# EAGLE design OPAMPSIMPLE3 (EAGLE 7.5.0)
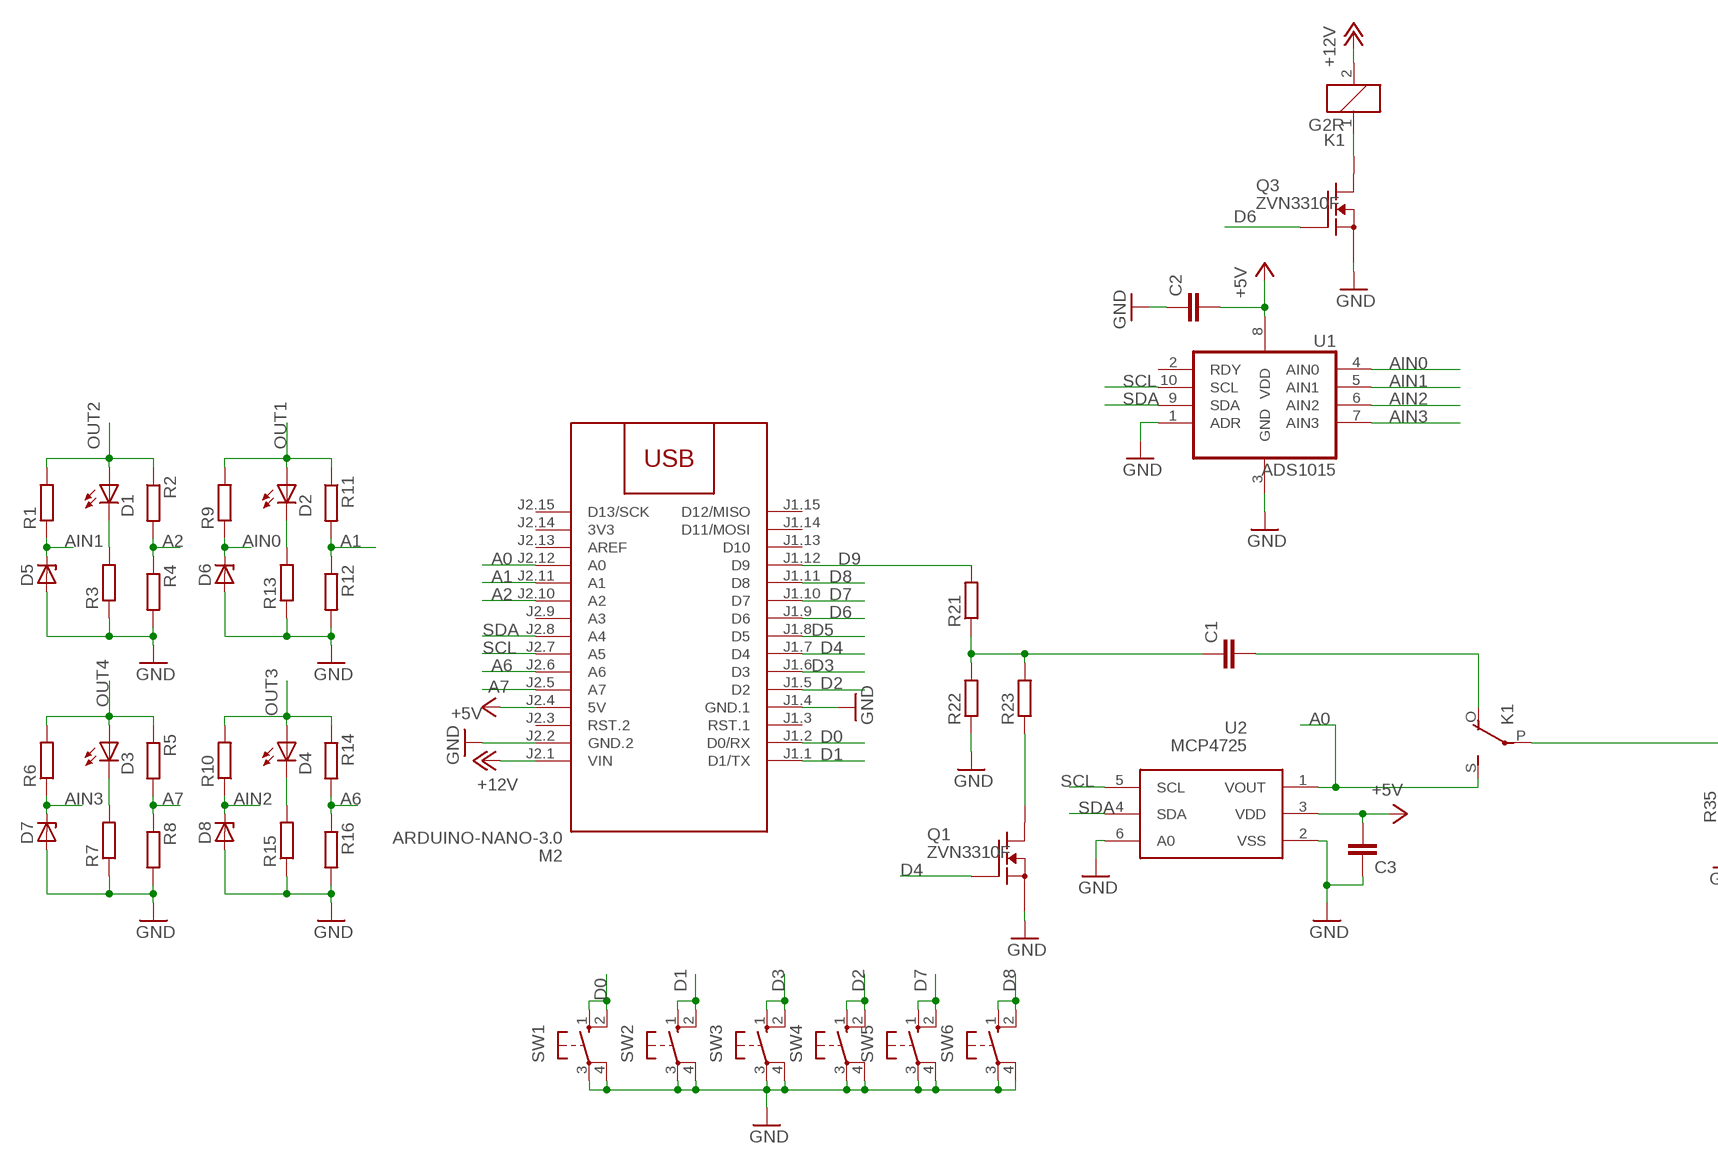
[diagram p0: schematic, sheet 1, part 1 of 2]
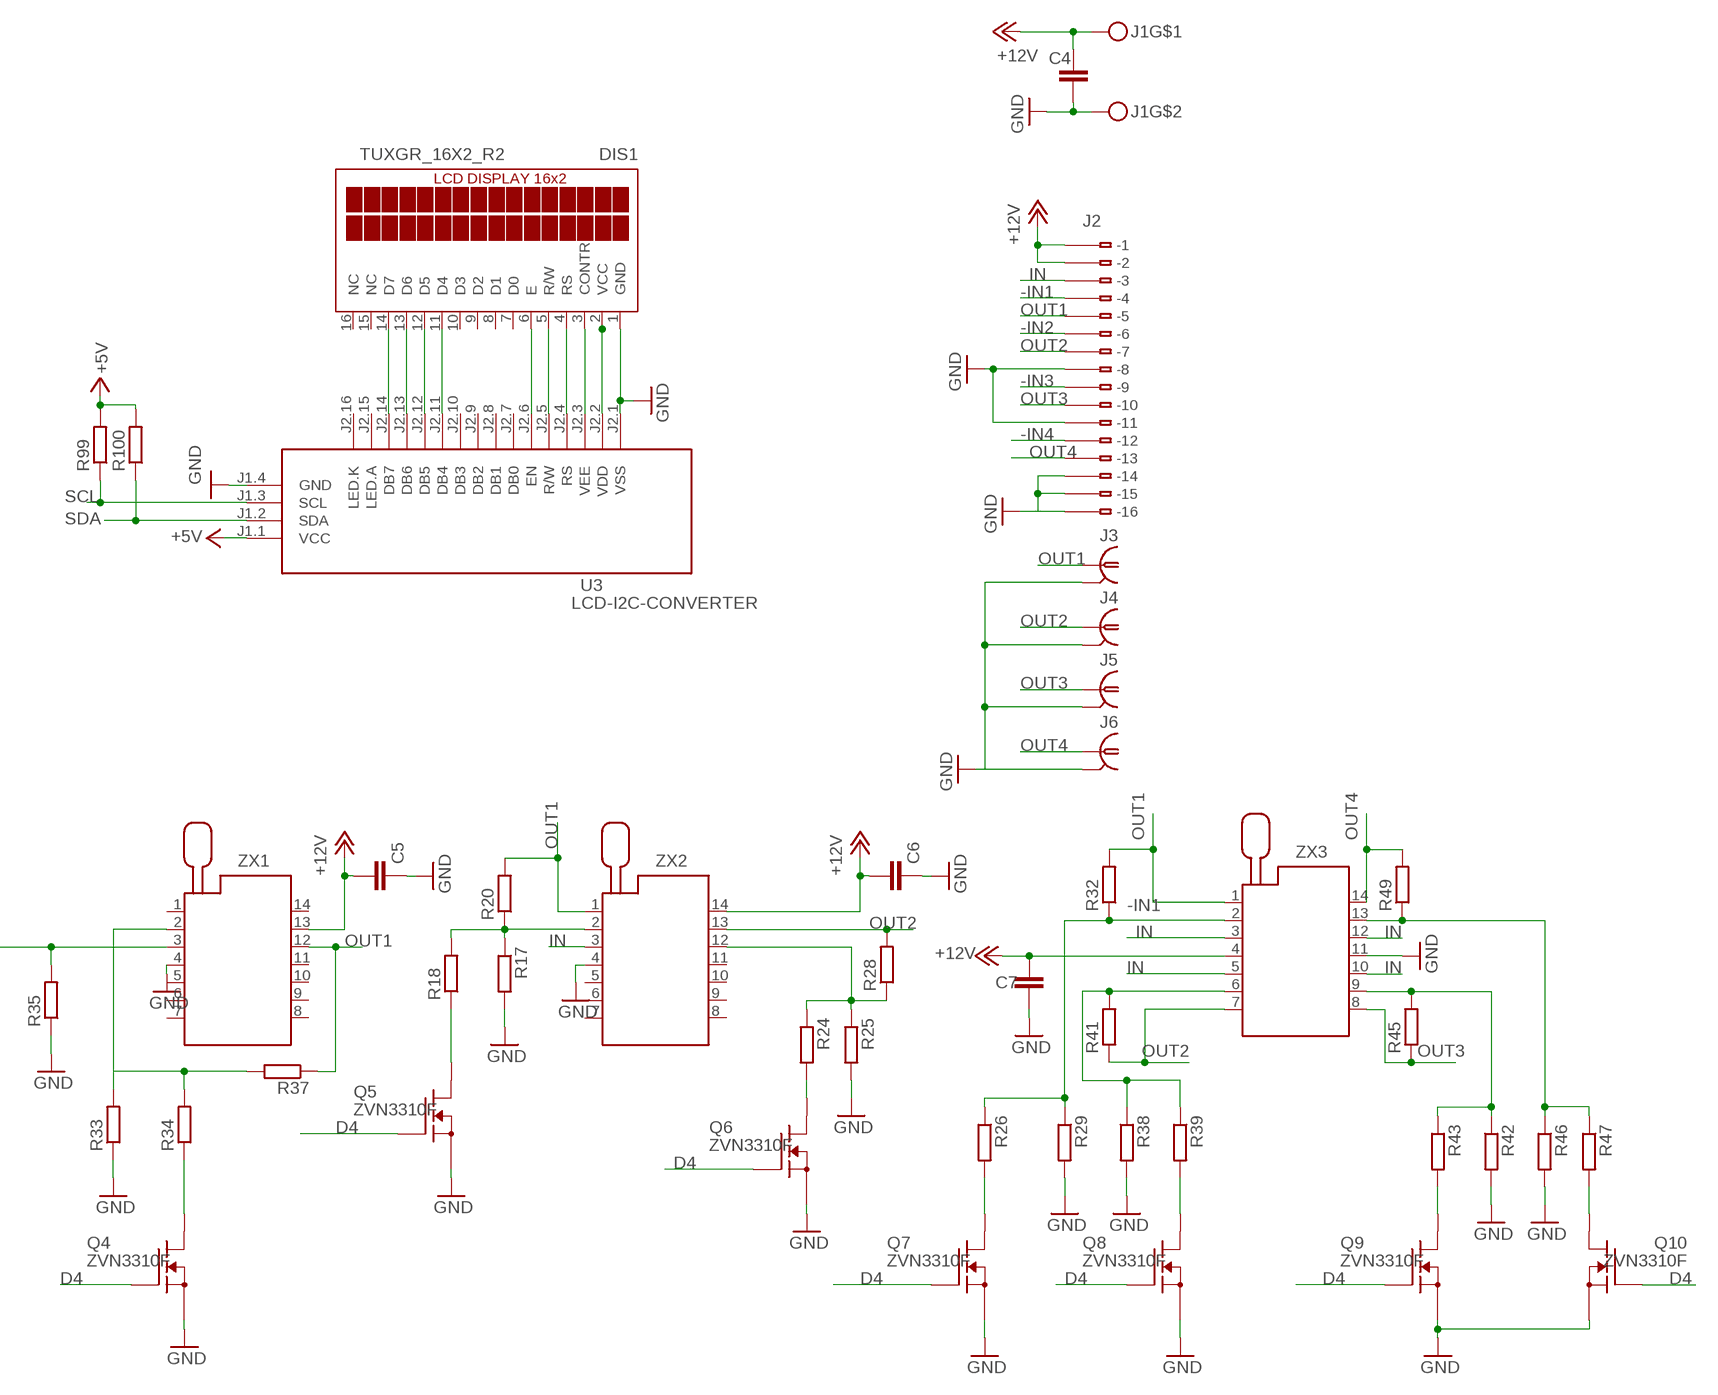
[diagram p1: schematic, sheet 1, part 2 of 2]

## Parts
C1  C-EUC1206  [C1206]
C2  C-EUC1206  [C1206]
C3  C-EUC1206  [C1206]
C4  C-EUC1206  [C1206]
C5  C-EUC1206  [C1206]
C6  C-EUC1206  [C1206]
C7  C-EUC1206  [C1206]
D1  LED5MM  [LED5MM]
D2  LED5MM  [LED5MM]
D3  LED5MM  [LED5MM]
D4  LED5MM  [LED5MM]
D5  BZX84CSMD  [TO236]
D6  BZX84CSMD  [TO236]
D7  BZX84CSMD  [TO236]
D8  BZX84CSMD  [TO236]
DIS1  TUXGR_16X2_R2  [TUXGR_16X2_R2]
J1  MKDSN1,5-2-5,08  [MKDSN1,5-2-5,08]
J2  233-116  [233-116]
J3  1-227161-0  [AMP_227161]
J4  1-227161-0  [AMP_227161]
J5  1-227161-0  [AMP_227161]
J6  1-227161-0  [AMP_227161]
K1  G2R  [G2R]
M2  ARDUINO-NANO-3.0  [ARDUINO-NANO-3.0]
Q1  ZVN3310F  BSS138  [SOT23]
Q3  ZVN3310F  BSS138  [SOT23]
Q4  ZVN3310F  BSS138  [SOT23]
Q5  ZVN3310F  BSS138  [SOT23]
Q6  ZVN3310F  BSS138  [SOT23]
Q7  ZVN3310F  BSS138  [SOT23]
Q8  ZVN3310F  BSS138  [SOT23]
Q9  ZVN3310F  BSS138  [SOT23]
Q10  ZVN3310F  BSS138  [SOT23]
R1  R-EU_R1206  [R1206]
R2  R-EU_R1206  [R1206]
R3  R-EU_R1206  [R1206]
R4  R-EU_R1206  [R1206]
R5  R-EU_R1206  [R1206]
R6  R-EU_R1206  [R1206]
R7  R-EU_R1206  [R1206]
R8  R-EU_R1206  [R1206]
R9  R-EU_R1206  [R1206]
R10  R-EU_R1206  [R1206]
R11  R-EU_R1206  [R1206]
R12  R-EU_R1206  [R1206]
R13  R-EU_R1206  [R1206]
R14  R-EU_R1206  [R1206]
R15  R-EU_R1206  [R1206]
R16  R-EU_R1206  [R1206]
R17  R-EU_R1206  [R1206]
R18  R-EU_R1206  [R1206]
R20  R-EU_R1206  [R1206]
R21  R-EU_R1206  [R1206]
R22  R-EU_R1206  [R1206]
R23  R-EU_R1206  [R1206]
R24  R-EU_R1206  [R1206]
R25  R-EU_R1206  [R1206]
R26  R-EU_R1206  [R1206]
R28  R-EU_R1206  [R1206]
R29  R-EU_R1206  [R1206]
R32  R-EU_R1206  [R1206]
R33  R-EU_R1206  [R1206]
R34  R-EU_R1206  [R1206]
R35  R-EU_R1206  [R1206]
R37  R-EU_R1206  [R1206]
R38  R-EU_R1206  [R1206]
R39  R-EU_R1206  [R1206]
R41  R-EU_R1206  [R1206]
R42  R-EU_R1206  [R1206]
R43  R-EU_R1206  [R1206]
R45  R-EU_R1206  [R1206]
R46  R-EU_R1206  [R1206]
R47  R-EU_R1206  [R1206]
R49  R-EU_R1206  [R1206]
R99  R-EU_R1206  [R1206]
R100  R-EU_R1206  [R1206]
SW1  40-XX  [B3F-40XX]
SW2  40-XX  [B3F-40XX]
SW3  40-XX  [B3F-40XX]
SW4  40-XX  [B3F-40XX]
SW5  40-XX  [B3F-40XX]
SW6  40-XX  [B3F-40XX]
U1  ADS1015  [ADS1015]
U2  MCP4725  [SOT23-6]
U3  LCD-I2C-CONVERTER  [LCD-I2C-CONVERTER]
ZX1  214-3339-00-0602J  [214-3339-00-0602J]
ZX2  214-3339-00-0602J  [214-3339-00-0602J]
ZX3  214-3339-00-0602J  [214-3339-00-0602J]

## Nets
+5V: C2.2 C3.2 M2.J2.4(5V) R99.2 R100.2 U1.8(VDD) U2.3(VDD) U3.J1.1(VCC)
+12V: C4.1 C5.2 C6.2 C7.1 J1.1 J2.B1(B-1) J2.B2(B-2) K1.2 M2.J2.1(VIN) ZX1.13 ZX2.14 ZX3.4
-IN1: J2.B4(B-4) R26.1 R29.1 R32.1 ZX3.2
-IN2: J2.B6(B-6) R38.1 R39.1 R41.2 ZX3.6
-IN3: J2.B9(B-9) R42.1 R43.1 R45.2 ZX3.9
-IN4: J2.B12(B-12) R46.1 R47.1 R49.1 ZX3.13
A0: K1.S(2:S) M2.J2.12(A0) U2.1(VOUT)
A1: M2.J2.11(A1) R11.2 R12.1
A2: M2.J2.10(A2) R2.2 R4.1
A6: M2.J2.6(A6) R14.2 R16.1
A7: M2.J2.5(A7) R5.2 R8.1
AIN0: D6.C R9.1 U1.4(AIN0)
AIN1: D5.C R1.1 U1.5(AIN1)
AIN2: D8.C R10.1 U1.6(AIN2)
AIN3: D7.C R6.1 U1.7(AIN3)
D0: M2.J1.2(D0/RX) SW1.1(S) SW1.2(S1)
D1: M2.J1.1(D1/TX) SW2.1(S) SW2.2(S1)
D2: M2.J1.5(D2) SW4.1(S) SW4.2(S1)
D3: M2.J1.6(D3) SW3.1(S) SW3.2(S1)
D4: M2.J1.7(D4) Q1.3(G) Q4.3(G) Q5.3(G) Q6.3(G) Q7.3(G) Q8.3(G) Q9.3(G) Q10.3(G)
D5: M2.J1.8(D5)
D6: M2.J1.9(D6) Q3.3(G)
D7: M2.J1.10(D7) SW5.1(S) SW5.2(S1)
D8: M2.J1.11(D8) SW6.1(S) SW6.2(S1)
D9: M2.J1.12(D9) R21.2
GND: C2.1 C3.1 C4.2 C5.1 C6.1 C7.2 D5.A D6.A D7.A D8.A DIS1.1(GND) J1.2 J2.B8(B-8) J2.B11(B-11) J2.B14(B-14) J2.B15(B-15) J2.B16(B-16) J3.2 J4.2 J5.2 J6.2 M2.J1.4(GND.1) M2.J2.2(GND.2) Q1.1(S) Q3.1(S) Q4.1(S) Q5.1(S) Q6.1(S) Q7.1(S) Q8.1(S) Q9.1(S) Q10.1(S) R3.1 R4.2 R7.1 R8.2 R12.2 R13.1 R15.1 R16.2 R17.2 R22.1 R25.2 R29.2 R33.1 R35.1 R38.2 R42.2 R46.2 SW1.3(P) SW1.4(P1) SW2.3(P) SW2.4(P1) SW3.3(P) SW3.4(P1) SW4.3(P) SW4.4(P1) SW5.3(P) SW5.4(P1) SW6.3(P) SW6.4(P1) U1.1(ADR) U1.3(GND) U2.2(VSS) U2.6(A0) U3.J1.4(GND) U3.J2.1(VSS) ZX1.4 ZX2.4 ZX3.11
IN: J2.B3(B-3) K1.P(2:P) R35.2 ZX1.3 ZX2.3 ZX3.3 ZX3.5 ZX3.10 ZX3.12
N$1: DIS1.14(D7) U3.J2.14(DB7)
N$2: DIS1.13(D6) U3.J2.13(DB6)
N$3: DIS1.12(D5) U3.J2.12(DB5)
N$4: DIS1.11(D4) U3.J2.11(DB4)
N$5: DIS1.6(E) U3.J2.6(EN)
N$6: DIS1.5(R/W) U3.J2.5(R/W)
N$7: DIS1.4(RS) U3.J2.4(RS)
N$8: C1.1 R21.1 R22.2 R23.2
N$10: DIS1.3(CONTR) U3.J2.3(VEE)
N$11: DIS1.2(VCC) U3.J2.2(VDD)
N$12: Q8.2(D) R39.2
N$13: R17.1 R18.2 R20.1 ZX2.2
N$14: K1.1 Q3.2(D)
N$15: R33.2 R34.2 R37.2 ZX1.2
N$16: C1.2 K1.O(2:O)
N$17: Q4.2(D) R34.1
N$18: Q5.2(D) R18.1
N$19: Q6.2(D) R24.2
N$20: D1.K(C) R3.2
N$21: Q7.2(D) R26.2
N$23: D2.K(C) R13.2
N$24: Q10.2(D) R47.2
N$25: Q9.2(D) R43.2
N$26: D3.K(C) R7.2
N$27: Q1.2(D) R23.1
N$29: D4.K(C) R15.2
N$32: R24.1 R25.1 R28.1 ZX2.12
OUT1: D2.A J2.B5(B-5) J3.1 R9.2 R11.1 R20.2 R32.2 R37.1 ZX1.12 ZX2.1 ZX3.1
OUT2: D1.A J2.B7(B-7) J4.1 R1.2 R2.1 R28.2 R41.1 ZX2.13 ZX3.7
OUT3: D4.A J2.B10(B-10) J5.1 R10.2 R14.1 R45.1 ZX3.8
OUT4: D3.A J2.B13(B-13) J6.1 R5.1 R6.2 R49.2 ZX3.14
SCL: M2.J2.7(A5) R99.1 U1.10(SCL) U2.5(SCL) U3.J1.3(SCL)
SDA: M2.J2.8(A4) R100.1 U1.9(SDA) U2.4(SDA) U3.J1.2(SDA)
Unconnected: DIS1.7(D0) DIS1.8(D1) DIS1.9(D2) DIS1.10(D3) DIS1.15(NC) DIS1.16(NC) J2.A1(-1) J2.A2(-2) J2.A3(-3) J2.A4(-4) J2.A5(-5) J2.A6(-6) J2.A7(-7) J2.A8(-8) J2.A9(-9) J2.A10(-10) J2.A11(-11) J2.A12(-12) J2.A13(-13) J2.A14(-14) J2.A15(-15) J2.A16(-16) M2.J1.3(RST.1) M2.J1.13(D10) M2.J1.14(D11/MOSI) M2.J1.15(D12/MISO) M2.J2.3(RST.2) M2.J2.9(A3) M2.J2.13(AREF) M2.J2.15(D13/SCK) U1.2(RDY) U3.J2.7(DB0) U3.J2.8(DB1) U3.J2.9(DB2) U3.J2.10(DB3) U3.J2.15(LED.A) U3.J2.16(LED.K) ZX1.1 ZX1.5 ZX1.6 ZX1.7 ZX1.8 ZX1.9 ZX1.10 ZX1.11 ZX1.14 ZX2.5 ZX2.6 ZX2.7 ZX2.8 ZX2.9 ZX2.10 ZX2.11

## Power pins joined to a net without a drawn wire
3V3: M2.J2.14(3V3)

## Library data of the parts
C1-C7 = rcl:C-EU: CAPACITOR, European symbol
D1-D4 = led:LED: LED
D5-D8 = diode:BZX84CSMD: Z DIODE
DIS1 = display-lcd:TUXGR_16X2_R2: Tuxgraphics LCD display 16x2 characters reflective, without background light Source: tuxgr_12x2_r2.pdf; OC_FARNELL: unknown; OC_NEWARK: unknown
J1 = con-phoenix-508:MKDSN1,5-2-5,08
J2 = con-wago:233-116: WAGO Cage Clamp; MPN: 233-116; OC_FARNELL: unknown; OC_NEWARK: 28K9054
J3-J6 = con-coax:?227161*: JACK, RIGHT ANGLE, 50 OHM, PCB, BNC; MF: TYCO ELECTRONICS; MPN: 1-227161; OC_FARNELL: unknown; OC_NEWARK: 33B3200
K1 = relay:G2R: RELAY 1 x switch, Omron; OC_FARNELL: 1569185; OC_NEWARK: unknown
M2 = diy-modules:ARDUINO-NANO-3.0: Arduino Nano 3.0 and compatible devices More details available here: https://www.arduino.cc/en/Main/ArduinoBoardNano Click here to find device on ebay.com
Q1 Q3-Q10 = transistor-fet:BSS138
R1-R18 R20-R26 R28 R29 R32-R35 R37-R39 R41-R43 R45-R47 R49 R99 R100 = rcl:R-EU_: RESISTOR, European symbol
SW1-SW6 = switch-omron:40-XX: OMRON SWITCH; MF: OMRON COMPONENTS USA; MPN: B3F-4000; OC_FARNELL: 176434; OC_NEWARK: 36K3105
U1 = burr-brown:ADS1015: 12BIT I2C DAC
U2 = linear:MCP4725
U3 = diy-modules:LCD-I2C-CONVERTER: I2C Bus to 4-Bit Parallel LCD Interface with LED backlight driver
ZX1-ZX3 = con-3m:214-3339-00-0602J: Zero Insertion Force Socked Source: http://www.3M.com/ehpd; MF: 3M; MPN: 214-3339-00-0602J; OC_FARNELL: 1247151; OC_NEWARK: 85K7793

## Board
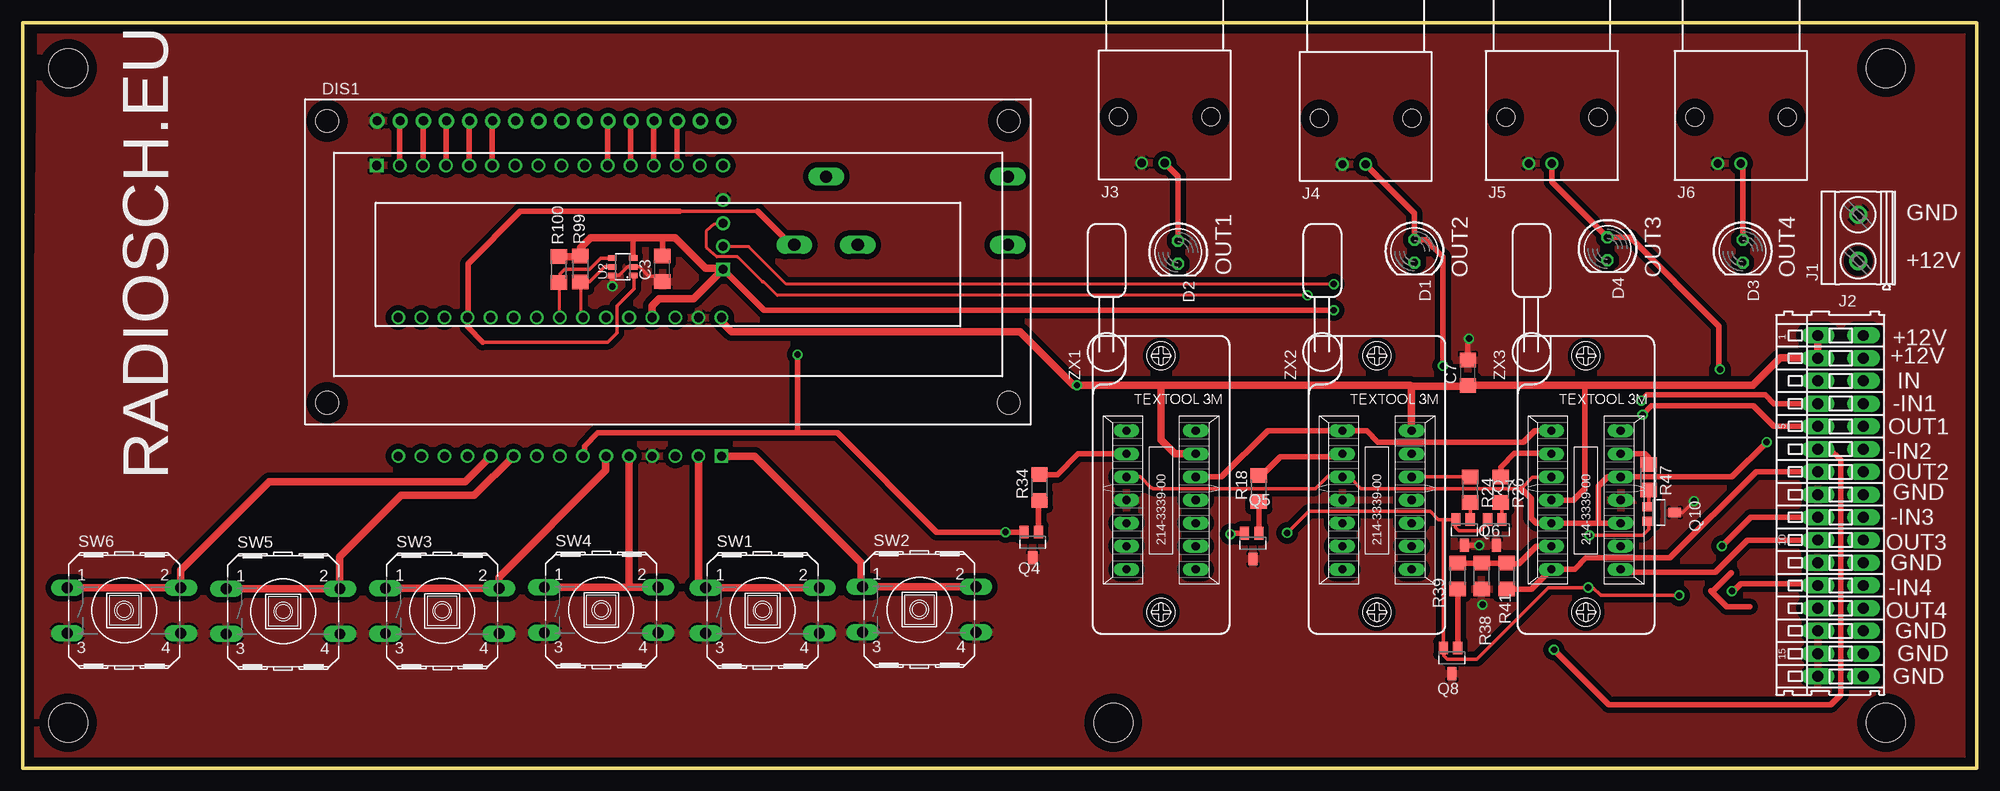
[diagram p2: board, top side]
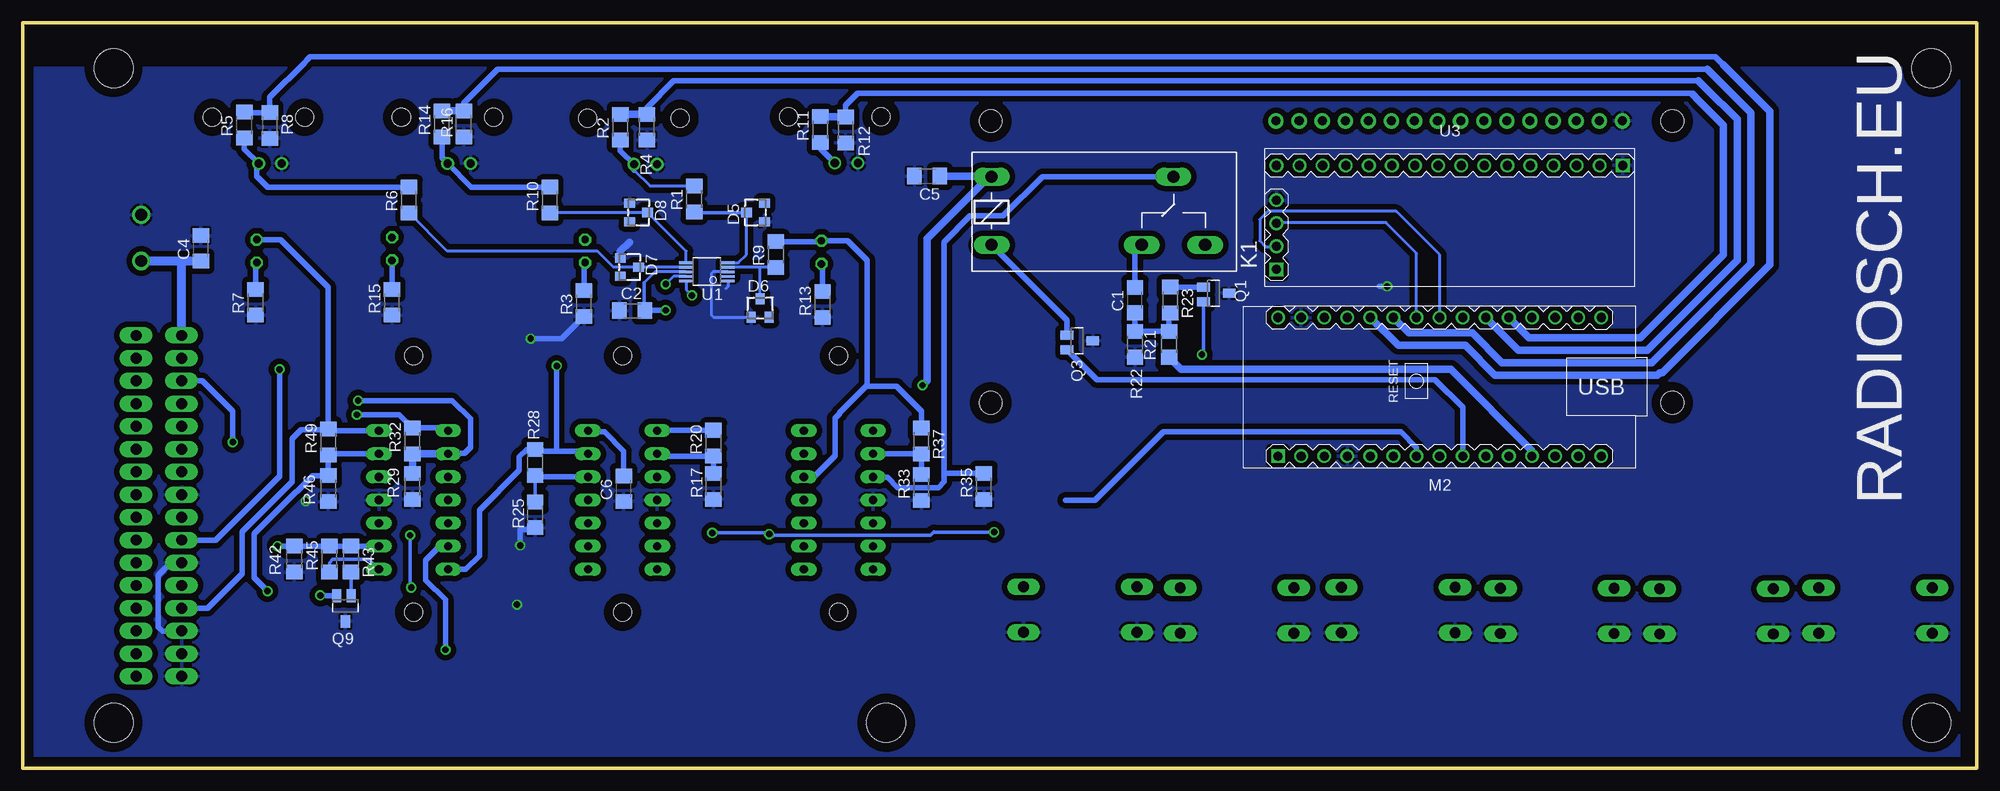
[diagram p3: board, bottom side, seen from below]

Size 215 x 82 mm. Coordinates in mm from the lower left corner, seen from the top.
Outline: 0,0 215,0 215,82 0,82 0,0
Copper layers (1*16): Top 0.035mm / dielectric 1.5mm / Bottom 0.035mm
Design rules "default": minimum track width 10mil, minimum drill 24mil, track to track 8mil, track to pad 8mil, pad to pad 8mil, via to via 8mil, smd to smd 8mil, copper to edge 40mil, drill to drill 8mil, minimum pad ring 10mil, minimum via ring 8mil, stop-mask expansion 4mil, vias tented up to drill 0mil, thermal gap 10mil
Holes 4.3 mm at 5,77 5,5 120,5 205,5 205,77

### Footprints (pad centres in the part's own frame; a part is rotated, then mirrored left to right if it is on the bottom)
C1206 = smd 1.6 x 1.8: 1 -1.4,0; 2 1.4,0
LED5MM = drill 0.813 octagon: A -1.27,0; K 1.27,0
TO236 = smd 1 x 1.2: A -1,-1; C 0,1; NC 1,-1
TUXGR_16X2_R2 = drill 1 pad 1.676: 1 -32,15.5; 2 -29.46,15.5; 3 -26.92,15.5; 4 -24.38,15.5; 5 -21.84,15.5; 6 -19.3,15.5; 7 -16.76,15.5; 8 -14.22,15.5; 9 -11.68,15.5; 10 -9.14,15.5; 11 -6.6,15.5; 12 -4.06,15.5; 13 -1.52,15.5; 14 1.02,15.5; 15 3.56,15.5; 16 6.1,15.5 | hole 2.5: -37.5,-15.5; 37.5,-15.5; -37.5,15.5; 37.5,15.5
MKDSN1,5-2-5,08 = drill 1.3 pad 2: 1 -2.561,0.025; 2 2.519,0.025
233-116 = drill 1.2 long: A1 -18.75,2.5; A2 -16.25,2.5; A3 -13.75,2.5; A4 -11.25,2.5; A5 -8.75,2.5; A6 -6.25,2.5; A7 -3.75,2.5; A8 -1.25,2.5; A9 1.25,2.5; A10 3.75,2.5; A11 6.25,2.5; A12 8.75,2.5; A13 11.25,2.5; A14 13.75,2.5; A15 16.25,2.5; A16 18.75,2.5; B1 -18.75,-2.5; B2 -16.25,-2.5; B3 -13.75,-2.5; B4 -11.25,-2.5; B5 -8.75,-2.5; B6 -6.25,-2.5; B7 -3.75,-2.5; B8 -1.25,-2.5; B9 1.25,-2.5; B10 3.75,-2.5; B11 6.25,-2.5; B12 8.75,-2.5; B13 11.25,-2.5; B14 13.75,-2.5; B15 16.25,-2.5; B16 18.75,-2.5
AMP_227161 = drill 0.9 pad 1.27: 1 0,-5.08; 2 -2.54,-5.08 | hole 2: -5.08,0; 5.08,0
G2R = drill 1.321 long: 1 -2.54,-3.683; 2 -2.54,3.81; O 13.97,-3.683; P 17.45,3.81; S 20.955,-3.683
ARDUINO-NANO-3.0 = drill 1 square: J1.1 17.78,7.62 | drill 1: J1.2 15.24,7.62; J1.3 12.7,7.62; J1.4 10.16,7.62; J1.5 7.62,7.62; J1.6 5.08,7.62; J1.7 2.54,7.62; J1.8 0,7.62; J1.9 -2.54,7.62; J1.10 -5.08,7.62; J1.11 -7.62,7.62; J1.12 -10.16,7.62; J1.13 -12.7,7.62; J1.14 -15.24,7.62; J1.15 -17.78,7.62; J2.1 17.78,-7.62; J2.2 15.24,-7.62; J2.3 12.7,-7.62; J2.4 10.16,-7.62; J2.5 7.62,-7.62; J2.6 5.08,-7.62; J2.7 2.54,-7.62; J2.8 0,-7.62; J2.9 -2.54,-7.62; J2.10 -5.08,-7.62; J2.11 -7.62,-7.62; J2.12 -10.16,-7.62; J2.13 -12.7,-7.62; J2.14 -15.24,-7.62; J2.15 -17.78,-7.62
SOT23 = smd 1 x 1.4: 1 0,1.735; 2 -0.632,-1.1; 3 0.95,-1.1
R1206 = smd 1.6 x 1.803: 1 -1.422,0; 2 1.422,0
B3F-40XX = drill 1.194 long: 1 -6.248,2.489; 2 6.248,2.489; 3 -6.248,-2.489; 4 6.248,-2.489
ADS1015 = smd 0.3 x 1.5: 1 -1.905,-2.616; 2 -1.405,-2.616; 3 -0.905,-2.616; 4 -0.405,-2.616; 5 0.095,-2.616; 6 0.095,1.984; 7 -0.405,1.984; 8 -0.905,1.984; 9 -1.405,1.984; 10 -1.905,1.984
SOT23-6 = smd 0.6 x 0.9: 1 -0.95,-1.15; 2 0,-1.15; 3 0.95,-1.15; 4 0.95,1.15; 5 0,1.15; 6 -0.95,1.15
LCD-I2C-CONVERTER = drill 1 square: J1.1 -19.05,-5.08; J2.1 19.05,6.35 | drill 1: J1.2 -19.05,-2.54; J1.3 -19.05,0; J1.4 -19.05,2.54; J2.2 16.51,6.35; J2.3 13.97,6.35; J2.4 11.43,6.35; J2.5 8.89,6.35; J2.6 6.35,6.35; J2.7 3.81,6.35; J2.8 1.27,6.35; J2.9 -1.27,6.35; J2.10 -3.81,6.35; J2.11 -6.35,6.35; J2.12 -8.89,6.35; J2.13 -11.43,6.35; J2.14 -13.97,6.35; J2.15 -16.51,6.35; J2.16 -19.05,6.35
214-3339-00-0602J = drill 0.9 long: 1 -7.62,-3.81; 2 -5.08,-3.81; 3 -2.54,-3.81; 4 0,-3.81; 5 2.54,-3.81; 6 5.08,-3.81; 7 7.62,-3.81; 8 7.62,3.81; 9 5.08,3.81; 10 2.54,3.81; 11 0,3.81; 12 -2.54,3.81; 13 -5.08,3.81; 14 -7.62,3.81 | hole 2: 12.35,0; -15.85,0

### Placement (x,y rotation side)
C1  92.62,51.5 90 bottom
C2  147.95,50.33 0 bottom
C3  70.38,54.92 90 top
C4  195.4,57.17 90 bottom
C5  115.5,65.12 0 bottom
C6  148.88,30.75 90 bottom
C7  159,43.5 90 top
D1  153.12,56.88 270 top
D2  127.12,56.75 270 top
D3  189.25,56.88 270 top
D4  174.38,57.12 270 top
D5  134.38,61.12 90 bottom
D6  133.88,50.62 0 bottom
D7  148.25,55.12 270 bottom
D8  147.25,61.12 270 bottom
DIS1  71,55.7 0 top
J1  201.97,58.35 90 top
J2  200.03,28.85 270 top
J3  125.65,71.65 0 top
J4  147.75,71.5 0 top
J5  168.25,71.6 0 top
J6  189.05,71.6 0 top
K1  105.85,61.25 0 bottom
M2  59.1,41.95 180 bottom
Q1  84,52.25 270 bottom
Q3  99,47 270 bottom
Q4  111.12,24.88 180 top
Q5  135.38,24.75 180 top
Q6  158.62,26.25 180 top
Q7  162.12,26.25 180 top
Q8  157.25,12.12 180 top
Q9  179.5,17.88 180 bottom
Q10  180,28.12 270 top
R1  141.12,62.62 90 bottom
R2  149.25,70.5 90 bottom
R3  153.25,51.12 90 bottom
R4  146.32,70.5 270 bottom
R5  190.62,70.75 90 bottom
R6  172.5,62.5 90 bottom
R7  189.38,51.25 90 bottom
R8  187.8,70.7 270 bottom
R9  132.12,56.5 90 bottom
R10  157,62.5 90 bottom
R11  127.25,70.25 90 bottom
R12  124.45,70.2 270 bottom
R13  127,51 90 bottom
R14  168.88,70.88 90 bottom
R15  174.38,51.25 90 bottom
R16  166.47,70.88 270 bottom
R17  139,31 270 bottom
R18  136,30.75 90 top
R20  139,35.75 90 bottom
R21  88.88,46.62 270 bottom
R22  92.62,46.62 90 bottom
R23  88.75,51.5 270 bottom
R24  159.25,30.62 270 top
R25  158.62,27.88 270 bottom
R26  162.62,30.62 270 top
R28  158.62,33.62 90 bottom
R29  172.12,31 270 bottom
R32  172.12,36 90 bottom
R33  116.12,30.88 90 bottom
R34  111.88,30.88 90 top
R35  109.25,31 90 bottom
R37  116.12,36 270 bottom
R38  160.5,21.12 270 top
R39  157.88,21.12 270 top
R41  163.25,21.12 90 top
R42  185.12,23 270 bottom
R43  178.88,23 270 bottom
R45  181.25,23 90 bottom
R46  181.38,30.75 270 bottom
R47  178.88,32 270 top
R49  181.38,35.88 90 bottom
R99  61.38,54.9 90 top
R100  59,54.85 90 top
SW1  81.4,17.35 0 top
SW2  98.65,17.45 0 top
SW3  46.15,17.3 0 top
SW4  63.65,17.4 0 top
SW5  28.65,17.25 0 top
SW6  11.15,17.35 0 top
U1  140.03,55.5 90 bottom
U2  66.03,55.15 90 top
U3  58,59.95 0 bottom
ZX1  125.25,29.5 270 top
ZX2  149,29.5 270 top
ZX3  172,29.5 270 top

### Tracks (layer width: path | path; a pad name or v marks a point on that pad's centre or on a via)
+5V  (via drill 0.7)
  Top 0.61: v144.25,50.38 81.55,50.38 U3.J1.1 | U2.3 67.17,58.3 67.25,58.38 | C3.2 70.38,58.38
  Top 0.813: R100.2 61.33,56.27 R99.2 61.38,57.25 62.5,58.38 67.25,58.38 70.38,58.38 71.75,58.38 75.12,55 76.92,55 U3.J1.1 73.81,51.62 70,51.62 69.26,50.89 M2.J2.4
  Bottom 0.305: U1.8 145.41,54.59 146.62,53.38 | 146.62,50.4 C2.2
  Bottom 0.406: 146.62,50.4 146.62,53.38
  Bottom 0.61: 146.62,50.4 144.28,50.4 v144.25,50.38
+12V  (via drill 0.7)
  Top 0.61: ZX3.4 170.62,29.5 171.88,30.75 171.88,42.12
  Top 0.813: M2.J2.1 76.88,49.12 78,48 109.75,48 115.62,42.12 v116,42.12 125.38,42.12 | 125.38,42.12 152.62,42.12 152.75,42 | ZX1.13 126.8,34.58 125.25,36.12 125.25,42 125.38,42.12 | 152.75,42 158.9,42 C7.1 171.85,42.1 171.88,42.12 190.38,42.12 193.38,45.12 197.5,45.12 J2.B2 J2.B1 | ZX2.14 152.81,41.94 152.75,42
  Bottom 0.61: C6.2 148.88,34.88 151,37 152.69,37 ZX2.14
  Bottom 0.813: v116,42.12 115.5,42.62 115.5,58.25 108.69,65.06 K1.2 108.58,65.25 109.12,65.25 109.25,65.12 C5.2
  Bottom 1.016: C4.1 197.88,55.78 | 197.88,55.78 201.94,55.78 J1.1 | J2.B1 197.53,55.42 197.88,55.78
-IN1  (via drill 0.7)
  Top 0.61: R26.1 162.62,33.12 164.12,34.62 168.15,34.62 ZX3.2 | J2.B4 192.67,40.1 191.72,41.05 178.71,41.05 v178.09,40.44
  Bottom 0.61: v178.09,40.44 167.73,40.44 165.71,38.41 165.71,35.28 166.37,34.62 168.15,34.62 ZX3.2
  Bottom 0.813: R29.1 R32.1 ZX3.2
-IN2  (via drill 0.7)
  Top 0.61: ZX3.6 166.54,24.42 164.62,22.5 163.3,22.5 R41.2 R38.1 R39.1 | J2.B6 198.84,35.1 200.03,33.91 200.03,8.05 198.93,6.96 174.54,6.96 v168.48,13.02
  Bottom 0.61: v168.48,13.02 168.48,18.52 170.66,20.7 170.66,22.88 169.12,24.41 168.21,24.41 ZX3.6
-IN3  (via drill 0.7)
  Top 0.61: J2.B9 190.12,27.6 v186.96,24.44
  Bottom 0.61: ZX3.9 180.75,24.42 | 180.75,24.42 R45.2 R42.1 185.14,24.44 v186.96,24.44 | R43.1 180.75,24.42
-IN4  (via drill 0.7)
  Top 0.61: R47.1 178.88,34.2 178.5,34.58 ZX3.13 | v188.07,19.48 188.24,19.48 189.03,20.28 197.34,20.28 J2.B12
  Bottom 0.61: ZX3.13 181.25,34.58 R49.1 R46.1 183.12,32.17 184.86,30.44 184.89,30.44 189.51,25.81 189.51,20.92 v188.07,19.48
A0
  Top 0.406: 50.62,46.88 64.38,46.88 65.38,47.88 65.38,50.88 67.25,52.75 67.25,54.12 U2.1 | 80.88,61.25 72.25,61.25
  Top 0.61: 50.62,46.88 48.94,48.56 M2.J2.12 49,49.63 49,55.5 54.75,61.25 72.25,61.25 | K1.S 84.56,57.57 80.88,61.25
A1
  Bottom 0.61: R12.1 124.45,72.92 123.12,74.25 31.38,74.25 30.62,73.5
  Bottom 0.813: 31.25,74.12 30.62,73.5 27.88,70.75 27.88,56.5 37,47.38 49.28,47.38 M2.J2.11 | R11.2 124.5,71.67 R12.1
A2
  Bottom 0.61: R4.1 146.32,72.67 143.38,75.62 30.62,75.62
  Bottom 0.813: 30.62,75.62 29.88,74.88 26.38,71.38 26.38,55.88 36.25,46 50.45,46 M2.J2.10 | R2.2 R4.1
A6
  Bottom 0.61: R16.1 166.47,73.15 162.75,76.88 29.62,76.88
  Bottom 0.813: 29.62,76.88 29.19,76.44 24.88,72.12 24.88,55.5 35.75,44.62 52.25,44.62 55.5,47.88 62.48,47.88 M2.J2.6 | R16.1 R14.2
A7
  Bottom 0.61: 190.57,72.12 R8.1 187.8,73.83 184,77.62 183.75,77.88 183.38,78.25 28.75,78.25 27.88,77.38
  Bottom 0.813: 27.88,77.38 22.75,72.25 22.75,55.38 34.62,43.5 34.88,43.5 35.12,43.25 53,43.25 56.25,46.5 63.65,46.5 M2.J2.5 | 190.57,72.12 R5.2
AIN0
  Bottom 0.305: R9.1 133.88,55.08 | 133.88,55.08 137.39,55.08 U1.4 | D6.C 133.88,55.08
AIN1
  Bottom 0.305: U1.5 136.28,55.59 135.38,56.5 D5.C
  Bottom 0.406: D5.C 141.05,61.12 R1.1
AIN2
  Bottom 0.305: R10.1 156.95,61.12 D8.C 142.01,56.88 U1.6
AIN3
  Bottom 0.305: U1.7 146.34,55.09 D7.C 150,55.12 151.75,56.88 168.3,56.88 R6.1
D0
  Top 0.813: M2.J1.2 74.34,20.65 SW1.1 SW1.2
D1
  Top 0.813: M2.J1.1 80.55,34.33 92.25,22.62 92.25,20.09 SW2.1 SW2.2
D2
  Top 0.813: SW4.1 66.5,19.89 | 66.5,19.89 SW4.2 | M2.J1.5 66.72,20.11 66.5,19.89
D3
  Top 0.813: M2.J1.6 64.12,34.27 64.12,32.75 52.4,21.02 SW3.2 SW3.1
D4  (via drill 0.7)
  Top 0.406: 156.12,27.35 Q6.3 157.62,27.3 157.62,26.5 158,26.12 160.38,26.12 161.18,26.92 Q7.3 | 156.12,27.35 155.78,27.35 154.88,28.25 141.5,28.25 v139.12,25.88 | 156.12,27.35 156.3,27.17 Q8.3 156.38,13.15 156.38,12.38 156.75,12 160,12 167.88,19.88 v172.25,19.88 172.75,19.88 173.62,19 v182.25,19 | Q10.3 178.9,26.27 178.25,25.62 v172.38,25.62 | 85.25,37 85,37
  Top 0.61: Q4.3 v108.12,25.98 100.53,25.98 89.62,36.88 85,36.88 | 85,36.88 63.25,36.88 61.81,35.44 61.81,34.5 M2.J1.7 | Q5.3 132.97,25.85 v132.88,25.75 | v85.25,45.5 85.25,37.12 | 85.25,37.12 85,36.88 | 85.25,37.12 85.25,37
  Bottom 0.406: 132.5,25.62 115.12,25.62 114.75,26 114.72,25.98 v108.12,25.98 | v139.12,25.88 133,25.88 v132.88,25.75 | v172.38,25.62 172.38,20 v172.25,19.88 | Q1.3 85.1,45.65 v85.25,45.5
  Bottom 0.61: M2.J1.7 61.64,35.27 63.38,37 89.5,37 97,29.5 100.28,29.5 | v132.88,25.75 132.62,25.75 132.5,25.62 | Q9.3 181.6,18.98 v182.25,19
D6
  Bottom 0.61: M2.J1.9 56.56,39.69 59.62,42.75 96.8,42.75 Q3.3
D7
  Top 0.813: M2.J1.10 49.69,30 41.62,30 34.9,23.27 SW5.2 SW5.1
D8
  Top 0.813: SW6.1 SW6.2 17.4,21.77 27.12,31.5 48.65,31.5 M2.J1.11
D9
  Bottom 0.61: 88.7,45.38 R21.2
  Bottom 0.813: M2.J1.12 48.94,34.94 57.88,43.88 87.55,43.88 R21.2
GND  (via drill 0.7)
  Top 0.406: U2.6 64.92,54.25 65.62,54.25 66.53,55.15 U2.2 67.85,55.15 68.88,54.12 69.78,54.12 C3.1 | Q10.1 182.62,28.12 v183.88,29.38
  Top 0.61: U2.6 v64.88,53 | C7.2 159,47.12 v159.12,47.25 | Q6.1 160.24,24.52 v160.25,24.5
  Bottom 0.305: U1.3 139.03,54.59 139.25,54.38 139.25,49.88 139,49.62 D6.A | U1.1 137.41,52.97 137.62,52.75
  Bottom 0.61: v64.88,53 65.75,53 | v159.12,47.25 155.7,47.25 R3.1 | v160.25,24.5 160.25,26.25 158.83,26.25 R25.2 | J2.B11 198.71,22.6 200.07,21.24 200.07,15.52 199.59,15.05 197.58,15.05 J2.B14
  Bottom 0.813: 158.88,26.2 R25.2 | D7.A 149.25,56.88 148.25,57.88
  other vias: 160.62,18
  pour Bottom (isolate 0.61): 2,77 219,77 219,1 2,1
  pour Top (isolate 0.61): 2,81 219,81 218,1 1,1
IN  (via drill 0.7)
  Top 0.406: ZX1.3 122.96,32.04 124.12,30.88 124.25,30.88 124.38,30.75 142.25,30.75 143.62,32.12 145.11,32.12 ZX2.3 145.96,32.04 147.25,30.75 164.88,30.75 166.12,32 168.15,32 ZX3.3
  Top 0.61: ZX3.10 173.5,26.96 | 173.5,26.96 ZX3.5 166.54,26.96 166,27.5 166,29.62 164.88,30.75 | 173.5,26.96 173.38,27.09 173.38,31 174.41,32.04 ZX3.12 188.04,32.04 v191.88,35.88
  Bottom 0.406: 168.15,32 ZX3.3
  Bottom 0.61: 113.62,32.38 113.62,57.88 110.75,60.75 107.12,60.75 102.81,65.06 K1.P 88.5,65.16 | 113.62,32.38 113.62,31.5 114.25,30.88 118.75,30.88 119.88,32 121.4,32 ZX1.3 | R35.2 113.58,32.42 113.62,32.38 | v191.88,35.88 191.88,39.25 195.25,42.62 197.5,42.62 J2.B3
N$1
  Top 0.61: U3.J2.14 71.97,71.15 DIS1.14
N$2
  Top 0.61: U3.J2.13 69.43,71.15 DIS1.13
N$3
  Top 0.61: U3.J2.12 66.89,71.15 DIS1.12
N$4
  Top 0.61: U3.J2.11 64.35,71.15 DIS1.11
N$5
  Top 0.61: U3.J2.6 51.65,71.15 DIS1.6
N$6
  Top 0.61: U3.J2.5 49.11,71.15 DIS1.5
N$7
  Top 0.61: U3.J2.4 46.57,71.15 DIS1.4
N$8
  Bottom 0.61: C1.1 R22.2 R21.1 88.88,49.95 R23.2
N$10
  Top 0.61: U3.J2.3 44.03,71.15 DIS1.3
N$11
  Top 0.61: U3.J2.2 41.49,71.15 DIS1.2
N$12
  Top 0.61: Q8.2 R39.2
N$13
  Top 0.61: R18.2 136.3,32.17 138.38,34.25 144.86,34.25 ZX2.2
  Bottom 0.61: R17.1 R20.1 144.94,34.33 ZX2.2
N$14
  Bottom 0.61: Q3.2 100.1,49.28 K1.1
N$15
  Top 0.61: R34.2 113.84,32.3 R37.2 ZX1.2
  Bottom 0.61: R33.2 R37.2 ZX1.2
N$16
  Bottom 0.61: C1.2 92.62,56.82 K1.O
N$17
  Top 0.61: Q4.2 111.76,29.34 R34.1
N$18
  Top 0.61: Q5.2 R18.1
N$19
  Top 0.406: Q6.2 R24.2
N$20
  Bottom 0.61: R3.2 153.25,55.48 D1.K
N$21
  Top 0.406: Q7.2 162.76,29.07 R26.2
N$22
  Top 0.61: 190,17.75 187.5,17.75 185.75,19.5 186,19.5 188,21.5
N$23
  Bottom 0.61: R13.2 127,55.36 D2.K
N$24
  Top 0.406: Q10.2 178.9,30.55 R47.2
N$25
  Bottom 0.406: R43.2 Q9.2
  Bottom 0.61: 178.87,21.57 R43.2
N$26
  Bottom 0.61: R7.2 189.38,55.48 D3.K
N$27
  Bottom 0.61: Q1.2 88.71,52.88 R23.1
N$29
  Bottom 0.61: R15.2 D4.K
N$32
  Top 0.406: R24.1 ZX2.12
  Bottom 0.406: R25.1 R28.1
  Bottom 0.61: ZX2.12 158.46,32.04 R28.1
OUT1  (via drill 0.7)
  Top 0.61: D2.A 127.12,65.09 J3.1 | ZX1.12 131.92,32.04 137,37.12 ZX2.1 147.88,37.12 149.12,35.88 165.12,35.88 166.38,37.12 ZX3.1 | J2.B5 192.65,37.6 190.4,39.85 179.21,39.85 v178.23,38.88
  Bottom 0.61: R9.2 127.22,57.92 D2.A 124.27,58.02 122.12,55.88 122.12,42.12 | 122.12,42.12 125.12,39.12 125.12,39 125.62,38.5 125.62,34.38 127.88,32.12 128.97,32.12 ZX1.12 | R37.1 116.12,39.25 118.88,42 122,42 122.12,42.12 | R20.2 145.14,37.17 ZX2.1 | ZX3.1 168.49,37.42 R32.2 173.58,38.88 v178.23,38.88 | 127.12,68.12 127.12,68.05 J3.1
  Bottom 0.813: 127.12,68.12 127.12,68.7 R11.1
OUT2  (via drill 0.7)
  Top 0.61: v156.25,44.25 156.25,56.25 154.35,58.14 D1.A 153.12,61.05 J4.1 | J2.B7 197.5,32.62 190.75,32.62 181.25,23.12 172,23.12 170.75,21.88 ZX3.7 166.01,19.7 R41.1
  Bottom 0.305: R1.2 146,64.05 147.75,65.8
  Bottom 0.61: ZX3.7 166.25,21.88 164.75,23.38 164.75,28.38 160.38,32.75 160.38,34.25 159.58,35.05 R28.2 157.92,35.05 157.75,34.88 156.25,34.88 | v156.25,44.25 156.25,34.88 | 156.25,34.88 153.1,34.88 ZX2.13 | 147.75,65.8 J4.1 149.25,67.92 R2.1
OUT3  (via drill 0.7)
  Top 0.61: J2.B10 189.75,25.1 186.23,21.58 176.11,21.58 ZX3.8 | v186.75,43.88 186.62,44 186.62,48.62 176.85,58.39 D4.A 168.25,64.52 J5.1
  Bottom 0.406: R45.1 181.25,22.62 180.88,23 176.93,23 ZX3.8
  Bottom 0.61: v186.75,43.88 186.75,32.1 193.75,25.1 J2.B10 | R10.2 165.65,63.92 J5.1 168.88,67.14 R14.1
OUT4
  Top 0.61: D3.A 189.25,66.32 J6.1
  Bottom 0.61: ZX3.14 181.2,37.12 R49.2 | R49.2 181.38,52.89 186.62,58.14 D3.A | J2.B13 194.65,17.6 190.88,21.38 190.88,26 185.38,31.5 185.38,36.25 184.38,37.25 181.42,37.25 R49.2 | R6.2 188.05,63.92 189.25,65.12 189.25,66.32 J6.1 190.62,68.09 R5.1
SCL  (via drill 0.7)
  Top 0.305: v141.38,52 83,52 81.5,53.5 81.38,53.5 78.62,56.25 76.38,56.25 75.25,57.25 75.25,59.12 76.12,59.88 76.97,59.88 U3.J1.3 | R99.1 61.38,49.83 M2.J2.7
  Top 0.406: U2.5 64.03,55.15 62.38,53.5 61.4,53.5 R99.1
  Bottom 0.305: U1.10 142.01,52.63 v141.38,52 | M2.J2.7 61.64,56.64 65,60 77,60 U3.J1.3
SDA  (via drill 0.7)
  Top 0.305: v144.25,53.25 84,53.25 79.88,57.38 77.09,57.38 U3.J1.2 | R100.1 59,49.67 M2.J2.8
  Top 0.406: U2.4 63.6,56.1 62.38,54.88 59.6,54.88 59.1,54.38 59.1,53.53 R100.1
  Bottom 0.305: U1.9 143.41,54.09 v144.25,53.25 | M2.J2.8 59.1,56.47 63.88,61.25 78,61.25 78.88,60.38 78.88,58 78.25,57.38 77.09,57.38 U3.J1.2

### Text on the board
tPlace: GND | +12V | OUT1 | OUT2 | OUT3 | OUT4 | +12V | +12V | IN | -IN1 | OUT1 | -IN2 | OUT2 | RADIOSCH.EU | GND | -IN3 | OUT3 | GND | -IN4 | OUT4 | GND | GND | GND
bPlace: RADIOSCH.EU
